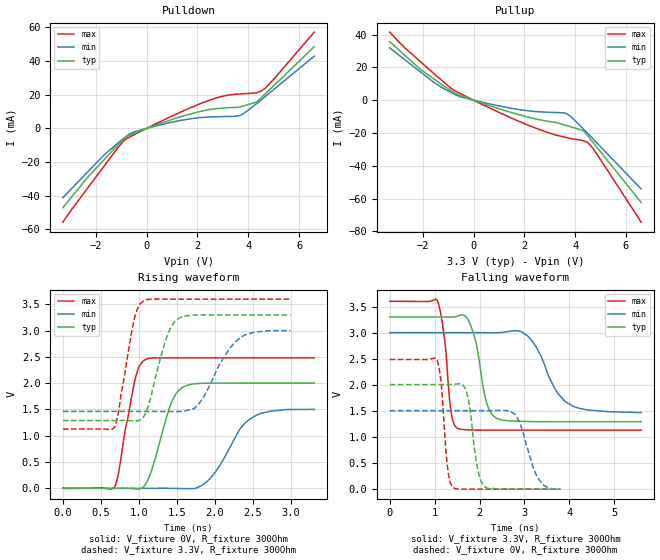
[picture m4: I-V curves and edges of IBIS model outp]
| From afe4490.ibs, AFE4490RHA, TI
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|   outp Model
[Model]   outp
Model_type   Output
Polarity   Non-Inverting
Vmeas = 1.65
Vref = 0
Cref = 2pF
Rref = 400
|   typ   min   max
|   (nom PVT)   (fast PVT)   (slow PVT)
C_comp   3.855e-13   3.543e-13   4.022e-13
| Where nom  PVT is Nominal Process, 3.3V, 27C
|   Fast PVT is Strong Process,  3.6V, -40C
|   Slow PVT is Weak Process,   3V, 105C
[Voltage Range]   3.3   3   3.6
|Junction Temperature
[Temperature Range]   27   105   -40
[Pullup Reference]   3.3   3   3.6
[Pulldown Reference]   0   0   0
[Power Clamp Reference]   3.3   3   3.6
[GND Clamp Reference]   0   0   0
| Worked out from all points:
|   slope of the pulldown table from 0 to 0.495 V, typ, clamps not added: 183 ohm
|   slope of the pullup table from 0 to 0.495 V, typ, clamps not added: 186 ohm
|   falling waveform, V_fixture 3.3V, R_fixture 300Ohm: 20-80 % time 254ps typ, 525ps min, 159ps max; typ from 3.3 V to 1.29 V
|   rising waveform, V_fixture 0V, R_fixture 300Ohm: 20-80 % time 242ps typ, 369ps min, 181ps max; typ from 0 V to 2 V
|   rising waveform, V_fixture 3.3V, R_fixture 300Ohm: 20-80 % time 224ps typ, 349ps min, 172ps max; typ from 1.29 V to 3.3 V
|   falling waveform, V_fixture 0V, R_fixture 300Ohm: 20-80 % time 179ps typ, 324ps min, 126ps max; typ from 2 V to 0 V
[Pulldown]
|   Voltage   I(typ)   I(min)   I(max)
-3.3V     -47.14mA   -41.14mA   -55.73mA
-2.307V   -28.73mA   -25.62mA   -35.12mA
-1.602V   -17.38mA   -14.79mA   -20.85mA
-896.4mV  -6.256mA   -5.74mA    -7.242mA
-504mV    -2.96mA    -2.116mA   -3.815mA
1.269V    6.595mA    4.579mA    9.214mA
2.833V    11.83mA    6.944mA    18.5mA
3.627V    12.53mA    7.489mA    20.43mA
4.316V    15.63mA    14.59mA    21.19mA
4.507V    18.17mA    16.93mA    22.17mA
4.968V    24.87mA    22.67mA    28.61mA
6.6V      48.57mA    42.93mA    57.21mA
[Pullup]
|   Voltage   I(typ)   I(min)   I(max)
-3.3V     35.71mA    31.82mA    41.49mA
-2.086V   18.73mA    17.15mA    23.38mA
-1.32V    10.26mA    8.373mA    12.96mA
-727.2mV  4.229mA    3.464mA    5.651mA
1.413V    -7.226mA   -4.782mA   -10.37mA
2.786V    -12.49mA   -7.293mA   -19mA
3.609V    -15.27mA   -7.947mA   -22.68mA
3.855V    -16.39mA   -10.47mA   -23.5mA
4.316V    -18.5mA    -17.43mA   -24.7mA
4.496V    -21.75mA   -20.28mA   -25.87mA
4.921V    -29.96mA   -27.12mA   -34.37mA
6.6V      -62.45mA   -54.19mA   -74.43mA
[Ramp]
R_load = 300
|   typ   min   max
dV/dt_r   1.20148/2.40176e-10   0.902117/3.68913e-10   1.4896/1.80585e-10
dV/dt_f   1.20465/2.50571e-10   0.921379/5.17237e-10   1.48167/1.58205e-10
[Falling Waveform]
V_fixture = 3.3V
V_fixture_min = 3V
V_fixture_max = 3.6V
R_fixture = 300Ohm
|   Time   V(typ)   V(min)   V(max)
0s        3.3V       3V         3.6V
1.056ns   3.3V       3V         3.616V
1.368ns   3.297V     3V         1.464V
1.524ns   3.321V     3V         1.159V
1.804ns   3.138V     3V         1.135V
2.162ns   1.64V      2.999V     1.13V
2.4ns     1.349V     2.999V     1.13V
3.062ns   1.296V     2.942V     1.131V
4.076ns   1.292V     1.59V      1.131V
5.598ns   1.292V     1.469V     1.131V
[Rising Waveform]
V_fixture = 0V
V_fixture_min = 0V
V_fixture_max = 0V
R_fixture = 300Ohm
|   Time   V(typ)   V(min)   V(max)
0s        3.925nV    10.51nV    3.294nV
678ps     12.5uV     2.546uV    14.32mV
958ps     -9.534mV   -31.57uV   2.116V
1.088ns   74.66mV    -4.034uV   2.449V
1.406ns   1.543V     505.9uV    2.482V
1.586ns   1.93V      -5.831mV   2.483V
1.948ns   2.001V     201.7mV    2.483V
2.32ns    2.002V     1.104V     2.483V
2.538ns   2.002V     1.385V     2.483V
3.31ns    2.002V     1.502V     2.483V
[Rising Waveform]
V_fixture = 3.3V
V_fixture_min = 3V
V_fixture_max = 3.6V
R_fixture = 300Ohm
|   Time   V(typ)   V(min)   V(max)
0s        1.291V     1.464V     1.128V
678ps     1.291V     1.464V     1.155V
946ps     1.285V     1.464V     3.254V
1.058ns   1.351V     1.464V     3.563V
1.35ns    2.802V     1.462V     3.6V
1.5ns     3.211V     1.462V     3.6V
1.792ns   3.3V       1.61V      3.6V
2.134ns   3.3V       2.529V     3.6V
2.358ns   3.3V       2.889V     3.6V
2.996ns   3.3V       3V         3.6V
[Falling Waveform]
V_fixture = 0V
V_fixture_min = 0V
V_fixture_max = 0V
R_fixture = 300Ohm
|   Time   V(typ)   V(min)   V(max)
0s        2.004V     1.504V     2.485V
1.044ns   2.004V     1.504V     2.491V
1.142ns   2.003V     1.504V     2.066V
1.286ns   2.003V     1.504V     423.8mV
1.398ns   2.006V     1.504V     39.31mV
1.702ns   1.889V     1.504V     -30.78uV
2.106ns   49.76mV    1.503V     -20.21uV
2.786ns   439.9uV    1.436V     -3.283uV
3.278ns   45.45uV    245.6mV    127.3nV
3.8ns     3.046uV    -939uV     43.03nV
